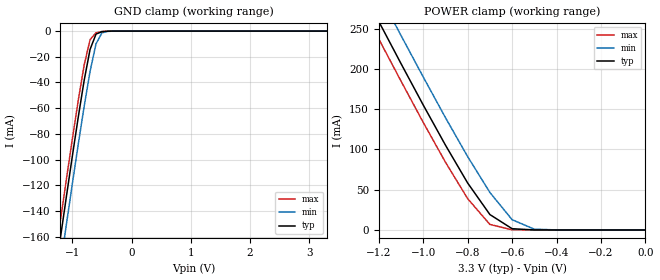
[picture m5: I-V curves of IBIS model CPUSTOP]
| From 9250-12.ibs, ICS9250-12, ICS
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|   Model CPUSTOP
[Model]   CPUSTOP
Model_type   Input
Polarity   Non-Inverting
Vinl = 800.00mV
Vinh =   2.00V
C_comp   5.50pF   5.00pF   6.00pF
[Temperature Range]   27.00   70.00   0.00
[Voltage Range]   3.30V   3.00V   3.70V
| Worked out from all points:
|   GND clamp passes 1 mA (typ) near -0.53 V on its own axis
|   POWER clamp passes 1 mA (typ) near -0.56 V on its own axis
[GND_clamp]
| voltage   I(typ)   I(min)   I(max)
-3.3V     -857mA     -877.7mA   -844.3mA
-1.3V     -193.1mA   -214.7mA   -179.6mA
-1.2V     -160.8mA   -182.5mA   -147.3mA
-1.1V     -128.9mA   -150.6mA   -115.5mA
-1V       -97.6mA    -119.1mA   -84.25mA
-900mV    -67.14mA   -88.3mA    -54.11mA
-800mV    -38.43mA   -58.65mA   -26.49mA
-700mV    -14.23mA   -31.32mA   -6.64mA
-600mV    -2.36mA    -9.93mA    -1.32mA
-500mV    -489.3uA   -1.38mA    -326.7uA
-400mV    -91.06uA   -228.9uA   -44.42uA
3.3V      108.9pA    1.5uA      48.42pA
[POWER_clamp]
| voltage   I(typ)   I(min)   I(max)
-3.3V     1.4A       1.43A      1.38A
-1.3V     311.6mA    346.5mA    289.9mA
-1.2V     258.8mA    293.7mA    237mA
-1.1V     206.5mA    241.4mA    184.8mA
-1V       155.1mA    189.9mA    133.5mA
-900mV    105.3mA    139.4mA    84.13mA
-800mV    58.26mA    91.04mA    38.85mA
-700mV    19.13mA    46.53mA    6.83mA
-600mV    1.55mA     12.75mA    234.8uA
-500mV    47.55uA    992.2uA    4.48uA
-400mV    1.09uA     42uA       71.42nA
0V        108.9pA    1.22nA     66.46pA
